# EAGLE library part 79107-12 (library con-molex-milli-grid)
RECEPTACAL
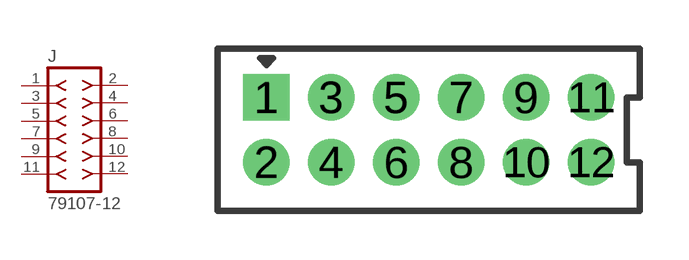
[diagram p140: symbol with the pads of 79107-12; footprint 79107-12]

Designator prefix J

## 79107-12  [79107-12]
1  1  pas
2  2  pas
3  3  pas
4  4  pas
5  5  pas
6  6  pas
7  7  pas
8  8  pas
9  9  pas
10  10  pas
11  11  pas
12  12  pas

## Footprint 79107-12 (pad centres in mm)
RECEPTACAL Dual Row, Vertical, Through-Hole
drill 0.914 square: 1 -5,1
drill 0.914: 2 -5,-1; 3 -3,1; 4 -3,-1; 5 -1,1; 6 -1,-1; 7 1,1; 8 1,-1; 9 3,1; 10 3,-1; 11 5,1; 12 5,-1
